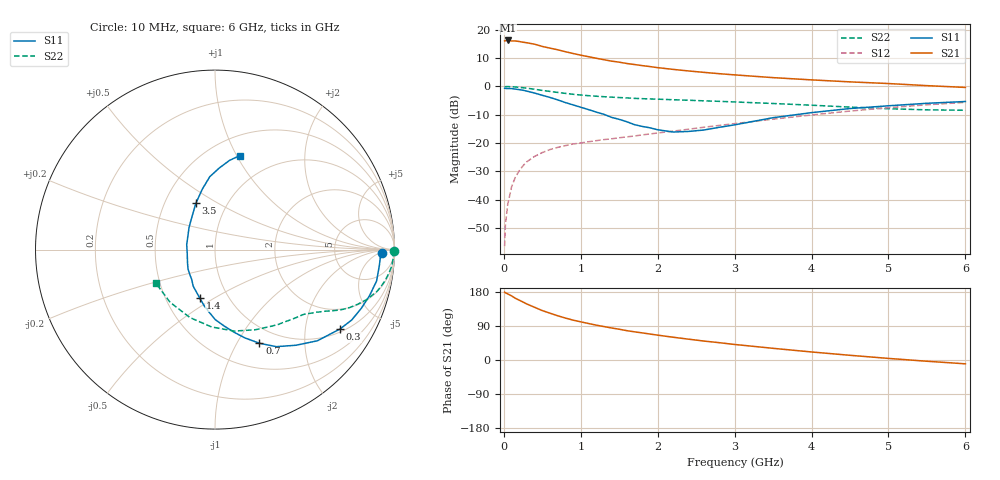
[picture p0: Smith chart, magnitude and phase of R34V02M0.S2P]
! SIEMENS Small Signal Semiconductors
! BFR181
! Si NPN RF Bipolar Junction Transistor in SOT23
! VCE = 4 V  IC = 2 mA
! Common Emitter S-Parameters:  May  1996
# GHz  S  MA  R  50
!  f  S11  S21  S12  S22
! GHz  MAG  ANG  MAG  ANG  MAG  ANG  MAG  ANG
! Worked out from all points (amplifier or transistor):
!   36 points, 10 MHz to 6 GHz, reference 50 ohm
!   highest |S21| = 16.3 dB at 50 MHz (marker M1)
!   |S21| within 3 dB of that: start of sweep to 649.4 MHz
!   unconditionally stable (mu >= 1): 1.613 GHz to 3.386 GHz
!   at 250 MHz: K = 0.23, MSG = 21.8 dB, |S12| = -28.0 dB
!   at 1.4 GHz: K = 0.94, MSG = 13.7 dB, |S12| = -18.5 dB
!   at 6 GHz: K = 0.86, MSG = 2.6 dB, |S12| = -5.6 dB
!   lowest NFmin = 1.35 dB at 450 MHz
!   S11 on the Smith chart (normalised r, x): 10 MHz: 25, -7; 300 MHz: 1.11, -3.09; 700 MHz: 0.79, -1.25; 1.4 GHz: 0.74, -0.43; 3.5 GHz: 0.71, +0.40; 6 GHz: 0.69, +1.03
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0.01  0.9282 -1.2  6.4 179.0  0.0015 87.6  0.9971 -0.5
0.02  0.923 -2.1  6.426 177.5  0.0035 89.1  0.9908 -1.1
0.05  0.9199 -5.6  6.506 174.5  0.0081 87.0  0.9943 -2.6
0.1  0.9172 -11.0  6.378 169.3  0.0167 82.6  0.9891 -5.2
0.15  0.8981 -16.7  6.371 162.9  0.0249 79.7  0.9771 -7.9
0.2  0.8783 -21.9  6.234 157.9  0.0323 76.9  0.9639 -10.2
0.3  0.8259 -32.3  5.917 147.7  0.0467 71.3  0.9315 -14.5
0.4  0.7638 -41.7  5.585 139.1  0.0581 66.6  0.8918 -18.1
0.5  0.6978 -49.8  5.1 130.4  0.0678 62.7  0.8508 -21.0
0.7  0.5777 -64.6  4.453 116.7  0.0837 57.7  0.7838 -25.2
0.8  0.5193 -71.3  4.115 110.7  0.0899 55.9  0.7542 -26.7
0.9  0.4719 -77.1  3.828 105.2  0.096 54.6  0.7277 -28.0
1.1  0.3901 -89.8  3.358 96.3  0.1052 53.7  0.6873 -30.2
1.2  0.3525 -95.0  3.155 92.0  0.11 53.2  0.6723 -31.2
1.4  0.2841 -107.3  2.805 84.5  0.1186 53.4  0.6471 -33.1
1.7  0.2109 -128.0  2.44 74.3  0.1332 54.4  0.6153 -35.7
2.2  0.1565 -171.4  2.004 60.1  0.1623 55.6  0.5826 -41.3
2.6  0.1697 152.6  1.775 50.0  0.1901 55.9  0.5569 -46.6
3.5  0.2803 112.3  1.432 30.8  0.264 53.3  0.4997 -63.4
4.5  0.4071 94.1  1.205 12.4  0.3672 45.3  0.4315 -92.5
5.5  0.5039 80.7  1.034 -3.3  0.474 32.9  0.3859 -130.4
6  0.5418 75.2  0.961 -10.1  0.5233 25.7  0.3793 -150.9
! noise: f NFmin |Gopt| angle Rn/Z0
0.45  1.35  0.6  17  0.4
0.9  1.45  0.5  36  0.4
1.8  1.8  0.31  80  0.37
